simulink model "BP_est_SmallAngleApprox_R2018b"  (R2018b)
settings: Solver=ode45  StartTime=0.0  StopTime=200  MaxStep=.01  MinStep=.0001  RelTol=1e-6  AbsTol=1e-6  EnableMultiTasking=on
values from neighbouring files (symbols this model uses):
  C = 0    [init_params.m]
  D = 0.11    [init_params.m]
  dtheta0 = 0    [init_params.m]
  h = 0.639    [init_params.m]
  I = 3.25e-4    (= 0.000325)    [init_params.m]
  KD = 0    [init_params.m]
  m = m_airplane + m_apparatus + m_ebox    (= 0.4714)    [init_params.m]
  theta0 = 0    [init_params.m]

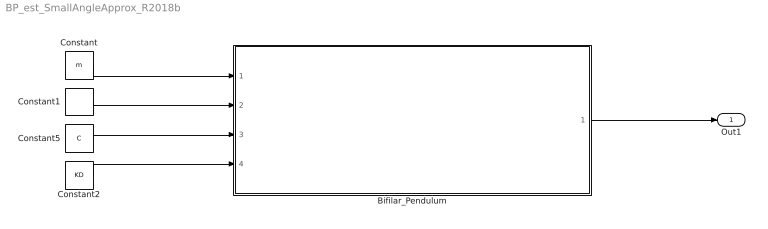
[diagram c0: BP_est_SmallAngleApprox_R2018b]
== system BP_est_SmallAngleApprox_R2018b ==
  Bifilar_Pendulum : Subsystem  mask(Bifilar Pendulum Simulation){D=D, SigD=0, h=h, Sigh=0, SigTh=0, ThSeed=0, TH0_THBIAS=theta0}
      mask prompts: D "Wire Displacement (D, meters)"; SigD "D Uncertainty (SigD, meters)"; h "Wire Height (h, meters)"; Sigh "h Uncertainty (Sigh, meters)"; SigTh "Theta Uncertainty (SigTh, radians)"; ThSeed "Theta Random Seed"; TH0_THBIAS "Initial Angular Displacement"
      mask help: This block simulates the response of a Bifilar Pendulum to an initial angular displacement. The parameters of the pendulum may be entered in the Mask Dialog.
  Constant : Constant  Value=m
  Constant1 : Constant  Value=I
  Constant2 : Constant  Value=KD
  Constant5 : Constant  Value=C
  Out1 : Outport
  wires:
  Constant/1 -> Bifilar_Pendulum/1(m)
  Constant1/1 -> Bifilar_Pendulum/2(I)
  Bifilar_Pendulum/1(theta) -> Out1/1
  Constant5/1 -> Bifilar_Pendulum/3(C)
  Constant2/1 -> Bifilar_Pendulum/4(KD)

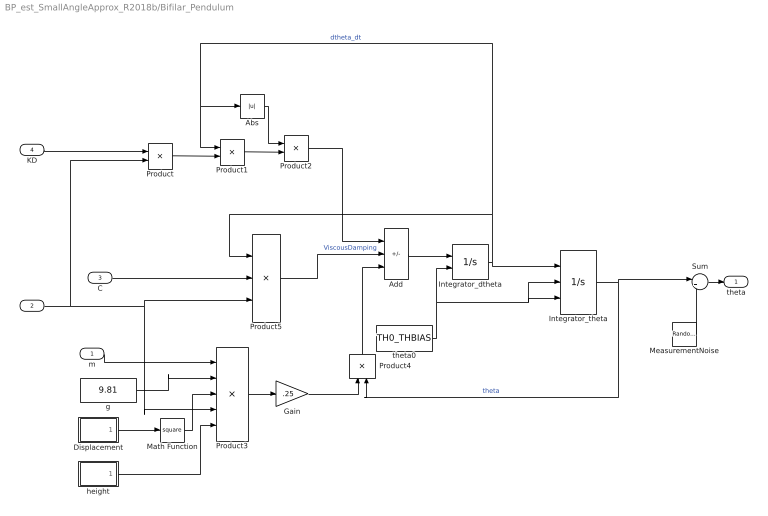
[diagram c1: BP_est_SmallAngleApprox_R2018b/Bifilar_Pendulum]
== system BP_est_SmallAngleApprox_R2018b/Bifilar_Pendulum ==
  m : Inport
  I : Inport  Port=2
  C : Inport  Port=3
  KD : Inport  Port=4
  Abs : Abs
  Add : Sum  Inputs=---
  Displacement : Subsystem
  Gain : Gain  Gain=.25
  Integrator_dtheta : Integrator  ExternalReset=either  InitialCondition=dtheta0
  Integrator_theta : Integrator  ExternalReset=either  InitialConditionSource=external
  Math Function : Math  Operator=square
  MeasurementNoise : RandomNumber  Variance=SigTh*SigTh  Seed=ThSeed  SampleTime=0
  Product : Product  Inputs=*/  RndMeth=Zero
  Product1 : Product  Inputs=**  RndMeth=Zero
  Product2 : Product  Inputs=**  RndMeth=Zero
  Product3 : Product  Inputs=***//  RndMeth=Zero
  Product4 : Product  Inputs=**  RndMeth=Zero
  Product5 : Product  Inputs=**/  RndMeth=Zero
  Sum : Sum  Inputs=|++
  g : Constant  Value=9.81
  height : Subsystem
  theta0 : Constant  Value=TH0_THBIAS
  theta : Outport
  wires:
  theta0/1 -> Integrator_dtheta/2, Integrator_theta/2, Integrator_theta/3
  Gain/1 -> Product4/1
  Product3/1 -> Gain/1
  height/1(h) -> Product3/5
  Math Function/1 -> Product3/3
  g/1 -> Product3/2
  m/1 -> Product3/1
  Displacement/1(D) -> Math Function/1
  Integrator_theta/1 -> Product4/2, Sum/1  "theta"
  Add/1 -> Integrator_dtheta/1
  C/1 -> Product5/2
  Product5/1 -> Add/2  "ViscousDamping"
  Product4/1 -> Add/3
  Sum/1 -> theta/1
  MeasurementNoise/1 -> Sum/2
  Product1/1 -> Product2/2
  Integrator_dtheta/1 -> Integrator_theta/1, Product5/1, Product1/1, Abs/1  "dtheta_dt"
  KD/1 -> Product/1
  Abs/1 -> Product2/1
  I/1 -> Product/2, Product5/3, Product3/4
  Product2/1 -> Add/1
  Product/1 -> Product1/2

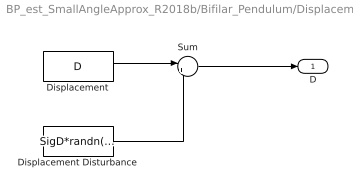
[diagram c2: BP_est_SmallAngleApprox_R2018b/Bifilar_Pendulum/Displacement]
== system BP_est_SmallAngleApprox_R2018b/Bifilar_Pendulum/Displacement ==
  Displacement : Constant  Value=D
  Displacement Disturbance : Constant  Value=SigD*randn(1)
  Sum : Sum  Inputs=|++
  D : Outport
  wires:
  Displacement Disturbance/1 -> Sum/2
  Sum/1 -> D/1
  Displacement/1 -> Sum/1

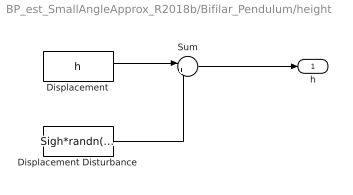
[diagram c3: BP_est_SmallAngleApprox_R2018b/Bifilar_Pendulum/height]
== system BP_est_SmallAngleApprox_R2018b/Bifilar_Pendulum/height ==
  Displacement : Constant  Value=h
  Displacement Disturbance : Constant  Value=Sigh*randn(1)
  Sum : Sum  Inputs=|++
  h : Outport
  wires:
  Displacement/1 -> Sum/1
  Sum/1 -> h/1
  Displacement Disturbance/1 -> Sum/2
